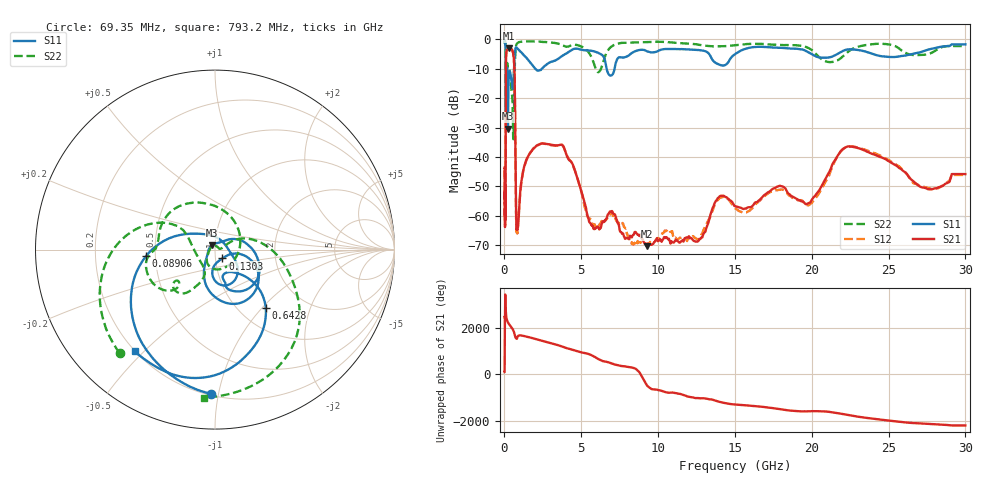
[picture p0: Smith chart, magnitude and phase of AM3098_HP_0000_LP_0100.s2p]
! Date/Time: Thu, Feb 28, 2019 8:30 AM
! Network Analyzer: Agilent Technologies E8364B Rev: A.07.50.67
! Sweep from 0.010 to 30.000 GHz, 1601 Points, Sweep Type: LOG
! Power Supply: 5.023 V, 0.002 A
# Hz S DB R 50
!freq MagS11 AngS11 MagS21 AngS21 MagS12 AngS12 MagS22 AngS22
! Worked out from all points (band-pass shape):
!   1601 points, 10 MHz to 30 GHz, reference 50 ohm
!   highest |S21| = -3.03 dB at 266.5 MHz (marker M1); lowest = -70.3 dB at 9.256 GHz (marker M2)
!   |S21| within 3 dB of the highest: 103.5 MHz to 601.5 MHz (498 MHz wide, 141 % of centre)
!   lowest |S11| = -30.4 dB at 227 MHz (marker M3), VSWR 1.06, Z = 48.1 + j2.29 ohm
!   |S11| at or under -10 dB: 176.1 MHz to 619 MHz (442.9 MHz wide, 111 % of centre); 2.013 GHz to 2.431 GHz (418.2 MHz wide, 18.8 % of centre); 6.649 GHz to 7.165 GHz (515.4 MHz wide, 7.46 % of centre)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
!   |S22| runs from -33.9 to -0.5 dB; largest |S21 - S12| = 0.013
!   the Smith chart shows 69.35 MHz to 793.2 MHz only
!   S11 on the Smith chart (normalised r, x): 69.35 MHz: 0.21, -0.95; 89.06 MHz: 0.44, -0.04; 130.3 MHz: 1.08, -0.11; 642.8 MHz: 1.32, -1.04; 793.2 MHz: 0.20, -0.47
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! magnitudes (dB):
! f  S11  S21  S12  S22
! 10 MHz  -0.3  -43.6  -44.3  -0.5
! 38.04 MHz  -0.5  -58.8  -60.0  -0.9
! 69.35 MHz  -1.9  -51.7  -53.8  -2.1
! 89.06 MHz  -8.3  -18.2  -18.1  -10.0
! 97.94 MHz  -24.2  -7.8  -7.8  -17.7
! 112.7 MHz  -13.6  -4.9  -4.9  -10.0
! 130.3 MHz  -23.9  -3.9  -3.8  -11.4
! 144.7 MHz  -13.1  -3.6  -3.5  -10.0
! 186.8 MHz  -11.5  -3.4  -3.4  -8.1
! 227 MHz  -30.4  -3.1  -3.1  -9.6
! 266.5 MHz  -14.6  -3.0  -3.0  -9.9
! 550.5 MHz  -16.8  -4.4  -4.3  -29.8
! 642.8 MHz  -7.4  -9.8  -9.7  -16.4
! 793.2 MHz  -2.8  -64.5  -64.7  -1.6
! 2.084 GHz  -10.4  -36.2  -36.3  -0.7
! 3.779 GHz  -5.5  -36.0  -36.0  -1.9
! 5.697 GHz  -3.9  -63.4  -62.3  -6.4
! 7.926 GHz  -5.9  -67.5  -64.2  -1.1
! 9.256 GHz  -4.0  -70.3  -69.5  -0.9
! 19.7 GHz  -4.1  -55.9  -56.4  -2.7
! 22.67 GHz  -3.4  -36.5  -36.4  -3.2
! 30 GHz  -1.7  -45.8  -46.1  -2.3
